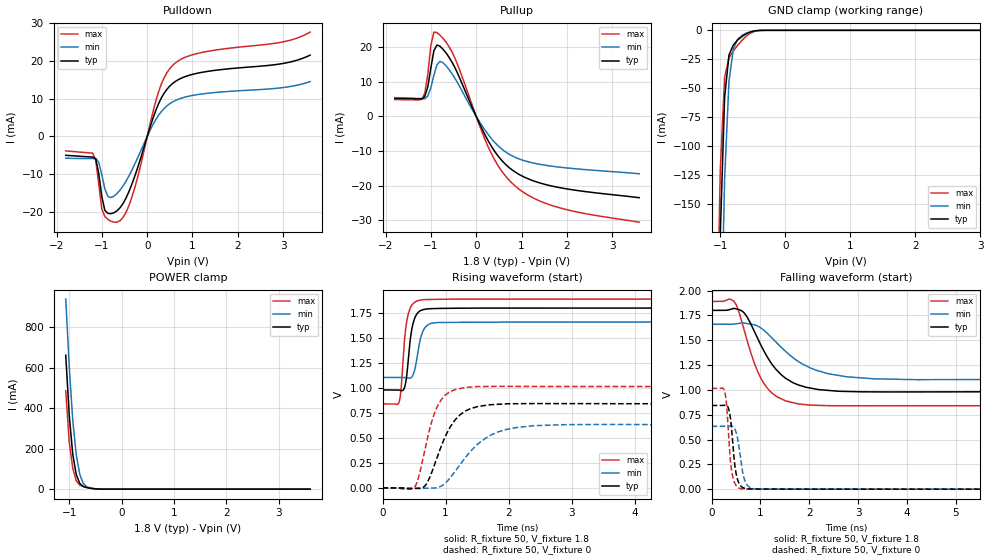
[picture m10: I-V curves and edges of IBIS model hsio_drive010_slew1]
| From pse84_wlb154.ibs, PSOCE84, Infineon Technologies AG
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[Model] hsio_drive010_slew1
Model_type I/O
Enable   Active-High
Vinl  =  0.54
Vinh  =  1.26
Vmeas =  0.9
Cref  =  15pF
| Capacitance   typ   min   max
C_comp   1.183861e-12   1.145095e-12   1.230403e-12
| Variables   typ   min   max
[GND Clamp Reference]   0   0   0
[POWER Clamp Reference]   1.8   1.66   1.89
[Pulldown Reference]   0   0   0
[Pullup Reference]   1.8   1.66   1.89
[Temperature Range]   25   125   -40
[Voltage Range]   1.8   1.66   1.89
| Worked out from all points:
|   slope of the pulldown table from 0 to 0.27 V, typ, clamps not added: 29.4 ohm
|   slope of the pullup table from 0 to 0.27 V, typ, clamps not added: 37.6 ohm
|   GND clamp passes 1 mA (typ) near -0.51 V on its own axis
|   POWER clamp passes 1 mA (typ) near -0.47 V on its own axis
|   falling waveform, R_fixture 50, V_fixture 1.8: 20-80 % time 615ps typ, 860ps min, 471ps max; typ from 1.8 V to 0.98 V
|   falling waveform, R_fixture 50, V_fixture 0: 20-80 % time 102ps typ, 122ps min, 91.8ps max; typ from 0.842 V to 0 V
|   rising waveform, R_fixture 50, V_fixture 1.8: 20-80 % time 92.9ps typ, 105ps min, 86.4ps max; typ from 0.98 V to 1.8 V
|   rising waveform, R_fixture 50, V_fixture 0: 20-80 % time 354ps typ, 555ps min, 257ps max; typ from 0 V to 0.842 V
[GND Clamp]
| Voltage   I(typ)   I(min)   I(max)
-1.137V   -688mA     -831.1mA   -596.4mA
-1.07V    -398.5mA   -545.5mA   -312.5mA
-1.003V   -176.8mA   -300mA     -120.9mA
-936.6mV  -57.93mA   -128.6mA   -40.51mA
-869.7mV  -21.44mA   -44.12mA   -23.78mA
-802.8mV  -12.54mA   -16.03mA   -17.79mA
-735.9mV  -8.37mA    -7.69mA    -12.93mA
-669mV    -5.28mA    -4.356mA   -8.606mA
-535.2mV  -1.316mA   -1.208mA   -2.332mA
-401.4mV  -73.56uA   -132.2uA   -119.3uA
3.6V      0A         0A         0A
[POWER Clamp]
| Voltage   I(typ)   I(min)   I(max)
-1.07V    662.2mA    940mA      485.7mA
-1.003V   363.7mA    605.6mA    233mA
-936.6mV  172.7mA    341mA      103.9mA
-869.7mV  72.74mA    168.6mA    41.65mA
-802.8mV  28.31mA    73.56mA    19.99mA
-735.9mV  13.11mA    28.55mA    13.36mA
-669mV    7.76mA     11.5mA     8.963mA
-535.2mV  2.357mA    2.863mA    2.668mA
-334.5mV  34.33uA    127.4uA    15.59uA
3.6V      0A         0A         0A
[Pulldown]
| Voltage   I(typ)   I(min)   I(max)
-1.8V     -5.002mA   -5.771mA   -3.816mA
-1.204V   -5.473mA   -5.879mA   -4.429mA
-1.137V   -5.945mA   -5.879mA   -6.426mA
-1.003V   -15.93mA   -10.12mA   -19.26mA
-869.7mV  -20.4mA    -15.91mA   -21.97mA
-602.1mV  -18.93mA   -14.24mA   -22.34mA
-468.3mV  -16.32mA   -11.87mA   -20.13mA
-267.6mV  -10.29mA   -7.131mA   -13.28mA
248.3mV   8.628mA    5.568mA    11.74mA
558.6mV   14.02mA    9.135mA    18.81mA
1.117V    16.78mA    11.11mA    22.02mA
3.6V      21.57mA    14.56mA    27.67mA
[Pullup]
| Voltage   I(typ)   I(min)   I(max)
-1.8V     5.223mA    5.46mA     4.891mA
-1.204V   5.078mA    5.172mA    4.961mA
-1.07V    8.58mA     5.916mA    12.21mA
-1.003V   13.97mA    8.283mA    20.49mA
-936.6mV  18.98mA    11.89mA    24.43mA
-869.7mV  20.69mA    14.95mA    24.31mA
-735.9mV  19.48mA    15.58mA    22.65mA
-468.3mV  14.06mA    11.02mA    16.81mA
310.3mV   -8.101mA   -5.989mA   -10.11mA
806.9mV   -15.59mA   -11.48mA   -19.48mA
1.738V    -20.32mA   -14.5mA    -26.03mA
3.6V      -23.51mA   -16.57mA   -30.6mA
[Ramp]
dV/dt_r   0.505345/0.354416n  0.379544/0.554567n  0.608663/0.256637n
dV/dt_f   0.49178/0.615168n  0.332578/0.860409n  0.629789/0.470568n
R_load = 50
[Falling Waveform]
R_fixture = 50
V_fixture = 1.8
V_fixture_min = 1.66
V_fixture_max = 1.89
| Time   V(typ)   V(min)   V(max)
0s        1.8V       1.66V      1.89V
492.2ps   1.817V     1.664V     1.867V
682.7ps   1.765V     1.672V     1.574V
878ps     1.585V     1.654V     1.265V
1.153ns   1.32V      1.563V     1.009V
1.512ns   1.117V     1.389V     889.5mV
2.009ns   1.019V     1.223V     846.7mV
2.75ns    983.7mV    1.132V     839.7mV
4.217ns   979.5mV    1.102V     840.4mV
50ns      980.4mV    1.106V     840.4mV
[Falling Waveform]
R_fixture = 50
V_fixture = 0
V_fixture_min = 0
V_fixture_max = 0
| Time   V(typ)   V(min)   V(max)
0s        842.2mV    632.6mV    1.014V
259.5ps   844.6mV    632.5mV    996mV
303.2ps   844.7mV    632.6mV    868.1mV
342ps     819mV      634.2mV    582.4mV
383.5ps   724.1mV    636.6mV    292mV
435.8ps   451.3mV    631mV      117.8mV
511.6ps   133.8mV    555.9mV    30.8mV
648.7ps   13.32mV    142.3mV    2.189mV
1.055ns   1.106mV    1.472mV    589.8uV
50ns      21.07nV    1.421uV    7.863nV
[Rising Waveform]
R_fixture = 50
V_fixture = 1.8
V_fixture_min = 1.66
V_fixture_max = 1.89
| Time   V(typ)   V(min)   V(max)
0s        980.4mV    1.106V     840.4mV
259.4ps   979.3mV    1.106V     854.4mV
293.4ps   974.2mV    1.106V     988mV
337.6ps   987.6mV    1.106V     1.402V
402.8ps   1.246V     1.099V     1.728V
444.4ps   1.509V     1.1V       1.807V
491.4ps   1.664V     1.142V     1.849V
600.2ps   1.774V     1.491V     1.88V
678.5ps   1.789V     1.609V     1.885V
50ns      1.8V       1.66V      1.89V
[Rising Waveform]
R_fixture = 50
V_fixture = 0
V_fixture_min = 0
V_fixture_max = 0
| Time   V(typ)   V(min)   V(max)
0s        21.14nV    1.417uV    7.861nV
493.1ps   -5.433mV   -2.729mV   91.43uV
648.8ps   6.702mV    -5.014mV   318mV
784.6ps   163.1mV    -2.044mV   675.5mV
928.4ps   413.5mV    16.62mV    881.2mV
1.15ns    680.6mV    164.8mV    984mV
1.49ns    810.7mV    427.2mV    1.014V
1.954ns   840.9mV    583.7mV    1.016V
2.848ns   843.5mV    632.8mV    1.014V
50ns      842.2mV    632.6mV    1.014V
